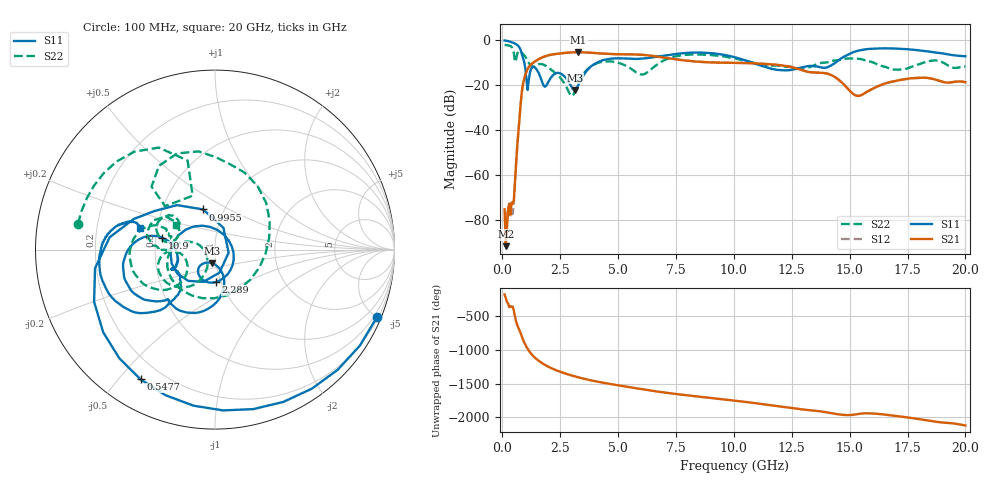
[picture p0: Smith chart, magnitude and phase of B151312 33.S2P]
!  2-Port S-parameters saved by WinCal
! VAR MeasName=S-Parameters (CALIBRATED_DATA) read from VNA (N5244A)
! VAR MeasDate=12/8/2015 5:46:06 PM
! VAR NAME=B151312 33
! VAR FILENAME=B151312 33.S2P
! VAR DATE=12/8/2015 5:46:06 PM
! VAR PHYS_PORTS=1,2
# Hz S DB R 50
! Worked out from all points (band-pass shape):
!   401 points, 100 MHz to 20 GHz, reference 50 ohm
!   highest |S21| = -5.42 dB at 3.284 GHz (marker M1); lowest = -91.6 dB at 149.8 MHz (marker M2)
!   |S21| within 3 dB of the highest: 1.588 GHz to 7.408 GHz (5.82 GHz wide, 129 % of centre)
!   lowest |S11| = -22.2 dB at 3.135 GHz (marker M3), VSWR 1.17, Z = 47.9 - j7.3 ohm
!   |S11| at or under -10 dB: 950.3 MHz to 4.092 GHz (3.142 GHz wide, 125 % of centre); 10.78 GHz to 14.39 GHz (3.615 GHz wide, 28.7 % of centre)
!   |S22| runs from -24.9 to -2.2 dB; largest |S21 - S12| = 0.0024
!   S11 on the Smith chart (normalised r, x): 100 MHz: 0.29, -4.99; 547.8 MHz: 0.12, -0.57; 995.5 MHz: 0.80, +0.38; 2.289 GHz: 0.95, -0.35; 10.9 GHz: 0.54, +0.08; 20 GHz: 0.40, +0.12
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1e8  -0.20 -22.6  -75.17 -175.5  -80.46 140.3  -2.19 169.3
1.4975e8  -0.28 -33.5  -91.55 136.9  -76.62 130.6  -2.23 163.9
3.985e8  -0.94 -87.2  -72.19 5.8  -74.75 9.4  -3.01 129.5
5.4775e8  -1.58 -119.8  -62.85 -142.3  -63.69 -150.0  -9.77 112.5
7.965e8  -4.57 173.3  -28.01 -32.5  -28.02 -32.5  -5.12 99.5
9.955e8  -12.64 106.5  -15.51 158.1  -15.51 158.1  -7.40 56.3
1.34375e9  -11.92 -162.3  -9.99 -12.8  -10.00 -12.8  -11.76 -58.0
1.692e9  -17.79 101.9  -7.88 -109.3  -7.89 -109.3  -10.69 -146.0
2.289e9  -14.87 -88.4  -6.22 144.0  -6.22 144.0  -14.61 166.9
3.13475e9  -22.23 -101.7  -5.43 47.8  -5.43 47.8  -22.88 -125.4
3.284e9  -20.04 -79.6  -5.42 33.9  -5.41 33.9  -19.25 -113.3
3.43325e9  -16.94 -72.7  -5.45 20.7  -5.44 20.7  -16.22 -113.9
4.9755e9  -8.11 -122.1  -6.29 -83.3  -6.29 -83.3  -10.00 -169.5
6.02025e9  -8.27 -133.9  -6.55 -141.7  -6.54 -141.8  -15.29 -159.8
6.7665e9  -7.28 -138.1  -7.48 179.1  -7.48 179.0  -10.28 -137.4
8.259e9  -5.59 -159.3  -9.47 115.9  -9.45 115.7  -6.46 -170.4
1.005e10  -7.68 171.0  -10.16 46.8  -10.15 46.7  -8.16 160.2
1.089575e10  -10.40 167.4  -10.35 11.0  -10.35 10.8  -10.22 157.2
1.338325e10  -11.50 -155.9  -14.41 -97.1  -14.40 -97.3  -11.66 -179.0
1.53235e10  -4.86 -142.6  -24.78 -154.3  -24.78 -154.4  -8.32 156.6
1.67165e10  -3.76 -172.5  -18.80 -167.7  -18.72 -168.6  -12.60 149.8
2e10  -7.22 163.6  -18.72 38.4  -18.77 38.0  -11.82 147.8
